INTERFACE I_Substate

METHOD PUBLIC IsEqual : BOOL
VAR_INPUT
	Substate : I_Substate;
END_VAR
END_METHOD

PROPERTY PUBLIC Name : T_MAXSTRING
GET
END_GET
END_PROPERTY

PROPERTY PUBLIC Next : I_Substate
GET
END_GET
SET
END_SET
END_PROPERTY

END_INTERFACE
